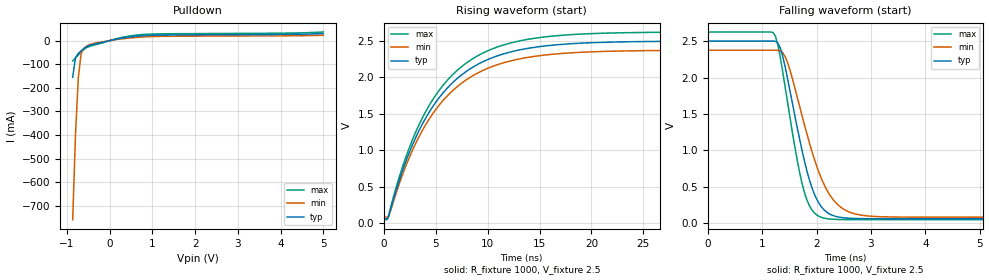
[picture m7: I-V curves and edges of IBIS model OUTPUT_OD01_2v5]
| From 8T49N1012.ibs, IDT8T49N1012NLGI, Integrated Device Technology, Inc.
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| 3.25758e+00   -2.18175e-02   -5.28494e-01   -1.12361e-02
| 3.33333e+00   -5.03221e-02   -7.41963e-01   -2.21762e-02
| 3.40909e+00   -2.62364e-01   -9.55797e-01   -3.46644e-02
| 3.48485e+00   -5.48353e-01   -1.16990e+00   -4.62641e-02
| 3.56061e+00   -8.34691e-01   -1.38422e+00   -9.04369e-02
| 3.63636e+00   -1.12135e+00   -1.59873e+00   -4.17088e-01
| 3.71212e+00   -1.40830e+00   -1.81343e+00   -7.83949e-01
| 3.78788e+00   -1.69551e+00   -2.02830e+00   -1.15114e+00
| 3.86364e+00   -1.98298e+00   -2.24333e+00   -1.51863e+00
| 3.93939e+00   -2.27067e+00   -2.45852e+00   -1.88638e+00
| 4.01515e+00   -2.55857e+00   -2.67387e+00   -2.25434e+00
| 4.09091e+00   -2.84666e+00   -2.88936e+00   -2.62250e+00
| 4.16667e+00   -3.13491e+00   -3.10499e+00   -2.99081e+00
| 4.24242e+00   -3.42332e+00   -3.32075e+00   -3.35927e+00
| 4.31818e+00   -3.71186e+00   -3.53663e+00   -3.72783e+00
| 4.39394e+00   -4.00052e+00   -3.75264e+00   -4.09651e+00
| 4.46970e+00   -4.28929e+00   -3.96875e+00   -4.46527e+00
| 4.54545e+00   -4.57816e+00   -4.18498e+00   -4.83412e+00
| 4.62121e+00   -4.86711e+00   -4.40130e+00   -5.20304e+00
| 4.69697e+00   -5.15613e+00   -4.61771e+00   -5.57201e+00
| 4.77273e+00   -5.44522e+00   -4.83422e+00   -5.94104e+00
| 4.84848e+00   -5.73437e+00   -5.05080e+00   -6.31011e+00
| 4.92424e+00   -6.02358e+00   -5.26747e+00   -6.67920e+00
| 5.00000e+00   -6.31282e+00   -5.48420e+00   -7.04832e+00
[Model] OUTPUT_OD01_2v5
Model_type   Open_drain
Polarity   Non-Inverting
|   typ   min   max
C_comp   2pF   1.5pF   2.5pF
Vmeas = 0.729V
Rref = 1000
Cref = 0
Vref = 2.5V
|   typ   min   max
[Voltage range]   2.5V   2.375V   2.625V
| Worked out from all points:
|   slope of the pulldown table from 0 to 0.375 V, typ, clamps not added: 28.6 ohm
|   rising waveform, R_fixture 1000, V_fixture 2.5: 20-80 % time 5.89ns typ, 5.96ns min, 5.83ns max; typ from 0.058 V to 2.5 V
|   falling waveform, R_fixture 1000, V_fixture 2.5: 20-80 % time 429ps typ, 552ps min, 357ps max; typ from 2.5 V to 0.058 V
[Pulldown]
|Note, modeling breaks down at 250mA and above.  This is well beyond the functional   |
|operating range of the device.  Should this scenario occur, catastrophic failure and   |
|possible damage to the device and/or board is of higher concern than the I-V curve   |
|behavior.  The IBIS checker will flag currents in excess of 10A with warnings.  Lines   |
|with currents in excess of 0.35 A have been commented out.  The points still remain|
|available to the user if the user desires to use them.   |
|Voltage   I (typ)   I (min)   I (max)
|-2.50000e+00   -1.22461e+01   -9.96179e+00   -1.48391e+01
|-2.20000e+00   -9.99080e+00   -8.26740e+00   -1.19637e+01
|-1.90000e+00   -7.73621e+00   -6.57432e+00   -9.08860e+00
|-1.60000e+00   -5.48288e+00   -4.88287e+00   -6.21429e+00
|-1.30000e+00   -3.23142e+00   -3.19335e+00   -3.34148e+00
|-1.00000e+00   -9.82636e-01   -1.50618e+00   -4.75877e-01
|-9.99000e-01   -9.75146e-01   -1.50057e+00   -4.67694e-01
|-9.32920e-01   -4.81499e-01   -1.12938e+00   -1.28883e-01
-866.8mV  -155.7mA   -758.5mA   -85.96mA
-800.8mV  -71.35mA   -397.8mA   -73.72mA
-734.7mV  -54.25mA   -156.2mA   -60.9mA
-668.6mV  -42.8mA    -55.01mA   -48.03mA
-602.5mV  -33.2mA    -32.01mA   -37.18mA
-536.4mV  -25.63mA   -22.78mA   -29.3mA
-338.2mV  -14.09mA   -10.49mA   -17.88mA
256.5mV   9.624mA    6.792mA    12.56mA
785.2mV   20.77mA    15.36mA    26mA
4.155V    26.3mA     20.4mA     31.86mA
5V        29.84mA    22.63mA    36.62mA
[Ramp]
|   typ   min   max
dV/dt_r   1.465/5.892n   1.377/5.96n   1.548/5.829n
dV/dt_f   1.465/0.429n   1.377/0.551n   1.548/0.357n
R_load =   50.0000
[Rising Waveform]
R_fixture = 1000
V_fixture = 2.5
V_fixture_min = 2.375
V_fixture_max = 2.625
C_fixture = 0.0p
| Time   typ   min   max
0s        58.29mV    79.84mV    46.07mV
311.1ps   57.79mV    78.84mV    47.72mV
488.9ps   110.1mV    101.3mV    127.2mV
2.356ns   935.8mV    869.4mV    1.001V
4.489ns   1.551V     1.456V     1.645V
6.933ns   1.969V     1.858V     2.08V
9.911ns   2.24V      2.119V     2.36V
13.33ns   2.386V     2.262V     2.51V
18.09ns   2.464V     2.339V     2.589V
40ns      2.5V       2.375V     2.625V
[Falling Waveform]
R_fixture = 1000
V_fixture = 2.5
V_fixture_min = 2.375
V_fixture_max = 2.625
C_fixture = 0.0p
| Time   typ   min   max
0s        2.5V       2.375V     2.625V
1.2ns     2.501V     2.375V     2.618V
1.289ns   2.473V     2.375V     2.45V
1.422ns   2.148V     2.287V     1.867V
1.778ns   850.6mV    1.348V     419.3mV
2ns       331.2mV    786.1mV    112.7mV
2.267ns   114.3mV    359.8mV    53.56mV
2.667ns   63.52mV    134.7mV    46.87mV
3.467ns   58.72mV    82.36mV    46.27mV
40ns      58.3mV     79.85mV    46.07mV
